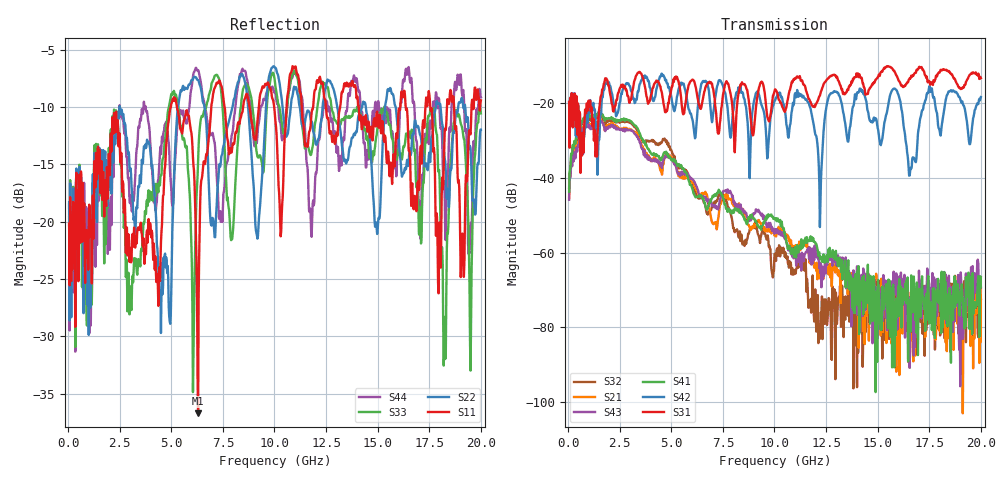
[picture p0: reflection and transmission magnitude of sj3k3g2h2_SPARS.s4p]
! FILE: E:\users\goganessyan\GBX_Backplane\FR408_backplane\1m_INBOUND_FEXT\sj3k3g2h2_SPARS.s4p
# MHZ S RI R 50.00
! FREQ  S11  S12  S13  S14
!  S21  S22  S23  S24
!  S31  S32  S33  S34
!  S41  S42  S43  S44
!  REAL  IMAG  REAL  IMAG  REAL  IMAG  REAL  IMAG
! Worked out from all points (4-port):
!   799 points, 50 MHz to 20 GHz, reference 50 ohm
!   strongest paths, dB at 50 MHz, 5.025 GHz, 10.03 GHz, 15.03 GHz, 20 GHz:
!     S31: -19.7, -15.6, -16.3, -12.9, -13.3
!     S42: -19.6, -19.2, -19.3, -27.2, -18.4
!     S41: -43.7, -35.0, -51.1, -67.3, -69.2
!     S43: -45.8, -35.2, -53.8, -75.2, -66.6
!     S21: -45.4, -34.6, -55.4, -68.4, -69.4
!     S32: -42.7, -32.9, -60.3, -73.9, -72.6
!   lowest |S11| = -36.7 dB at 6.3 GHz (marker M1), VSWR 1.03, Z = 48.6 - j0.109 ohm
!   |S11| at or under -10 dB: start of sweep to 4.978 GHz; 5.273 GHz to 6.939 GHz (1.666 GHz wide, 27.3 % of centre); 14.08 GHz to 16.1 GHz (2.017 GHz wide, 13.4 % of centre)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
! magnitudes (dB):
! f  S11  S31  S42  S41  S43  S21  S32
! 50 MHz  -20.2  -19.7  -19.6  -43.7  -45.8  -45.4  -42.7
! 6.3 GHz  -36.7  -19.3  -20.3  -45.1  -43.4  -44.1  -45.4
! 11.35 GHz  -11.0  -14.0  -18.4  -58.8  -61.5  -58.0  -62.8
! 12.2 GHz  -7.3  -18.0  -53.2  -61.7  -62.8  -66.9  -83.1
! 12.88 GHz  -12.5  -12.4  -16.8  -61.5  -61.1  -64.5  -74.8
! 16.57 GHz  -14.7  -13.4  -38.2  -72.7  -72.1  -73.5  -76.9
! 20 GHz  -9.4  -13.3  -18.4  -69.2  -66.6  -69.4  -72.6
